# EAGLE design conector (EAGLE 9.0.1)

## Sheet 1 of 2: Board to Board Headers
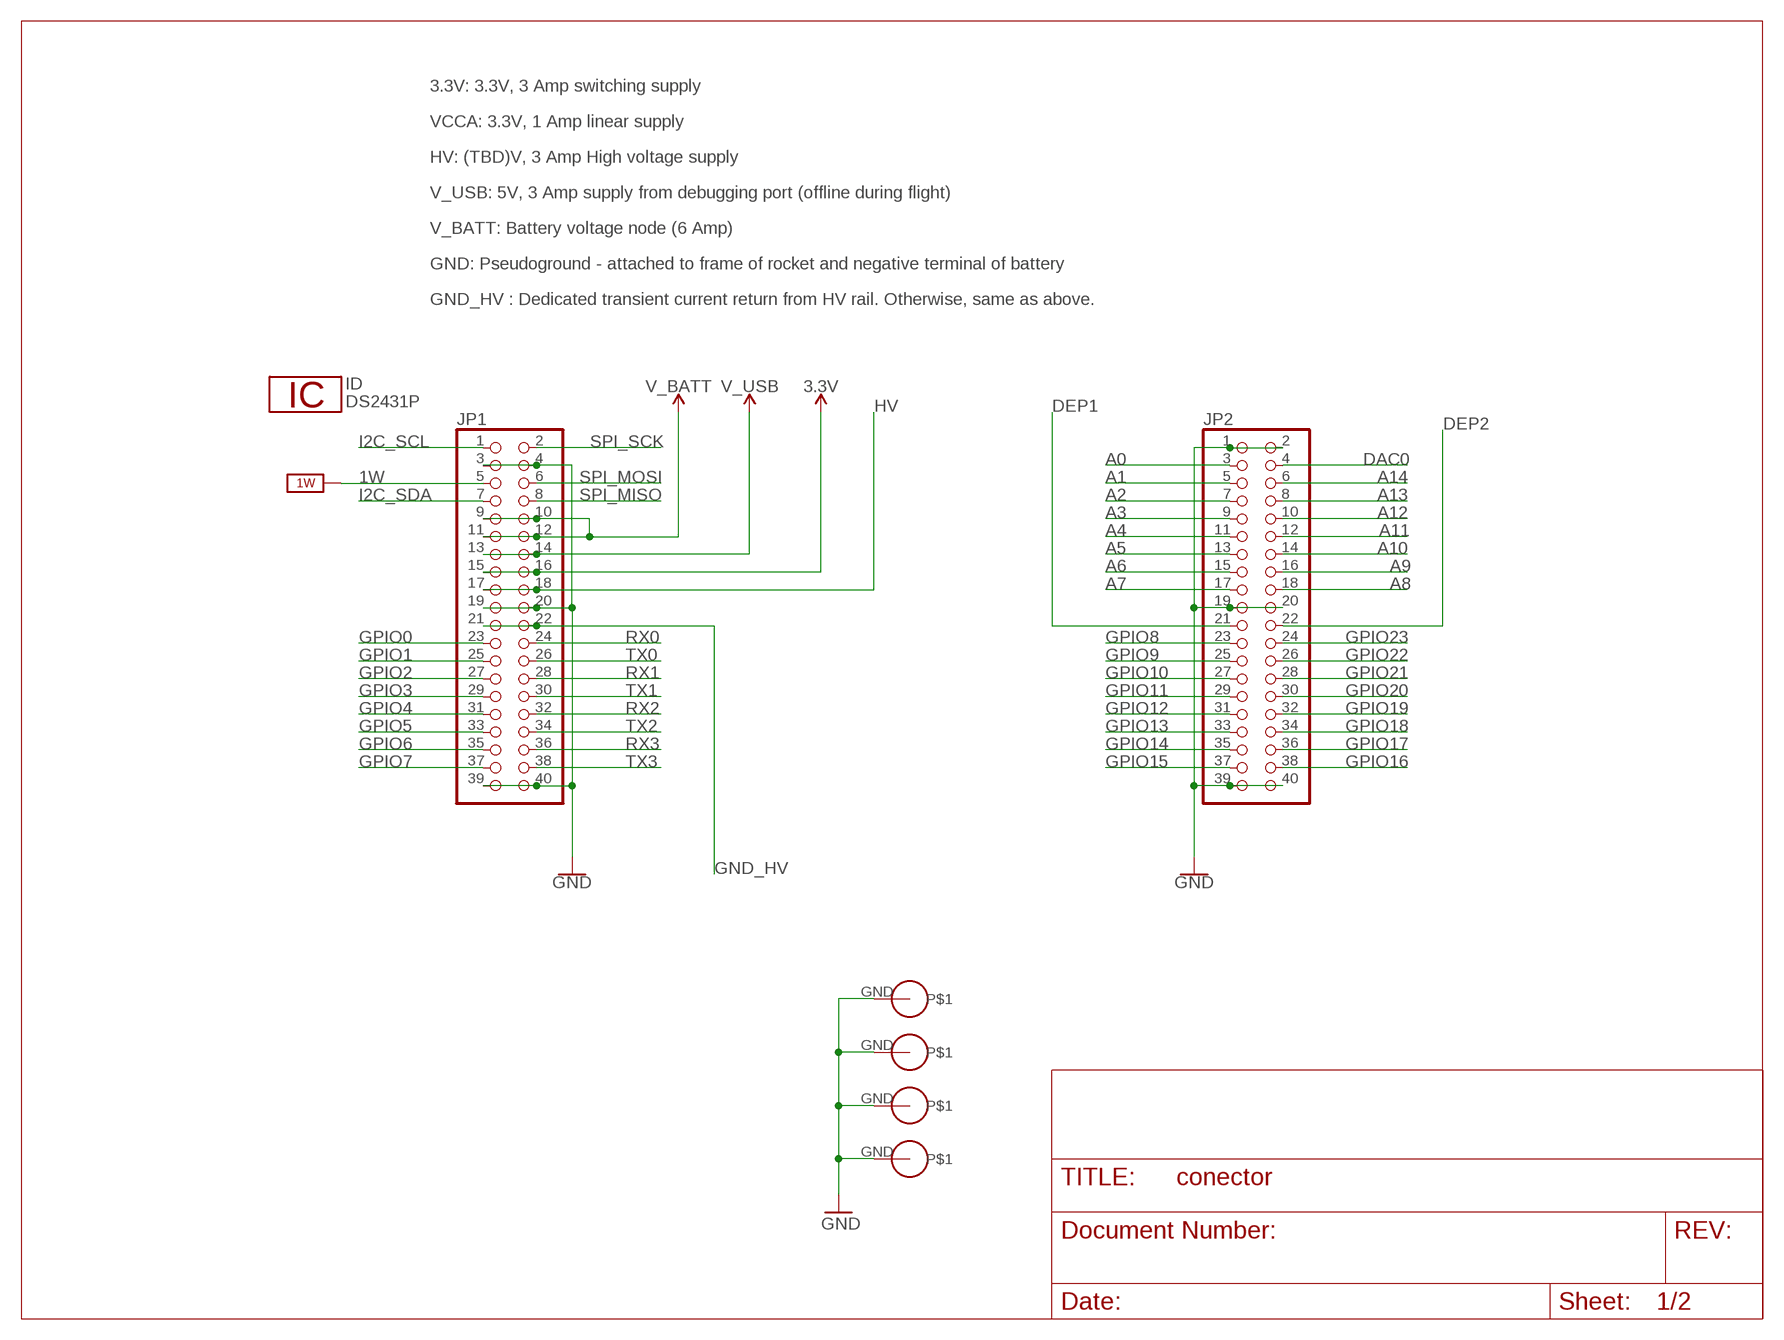
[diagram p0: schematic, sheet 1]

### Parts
ID  DS2431P  [TSOC6]
JP1  PINHD-2X20  [2X20]
JP2  PINHD-2X20  [2X20]
U$1  PS/104-MOUNTING-HOLE  [PC/104-MOUNTING-HOLE]
U$2  PS/104-MOUNTING-HOLE  [PC/104-MOUNTING-HOLE]
U$3  PS/104-MOUNTING-HOLE  [PC/104-MOUNTING-HOLE]
U$4  PS/104-MOUNTING-HOLE  [PC/104-MOUNTING-HOLE]

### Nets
1W: JP1.5 ; supply symbol labelled 1W_SUP
3.3V: JP1.15 JP1.16 ; also sheet 2
A0: JP2.3
A1: JP2.5
A2: JP2.7
A3: JP2.9
A4: JP2.11
A5: JP2.13
A6: JP2.15
A7: JP2.17
A8: JP2.18
A9: JP2.16
A10: JP2.14
A11: JP2.12
A12: JP2.10
A13: JP2.8
A14: JP2.6
DAC0: JP2.4
DEP1: JP2.21 ; also sheet 2
DEP2: JP2.22 ; also sheet 2
GND: JP1.3 JP1.4 JP1.19 JP1.20 JP1.39 JP1.40 JP2.1 JP2.2 JP2.19 JP2.20 JP2.39 JP2.40 U$1.GND U$2.GND U$3.GND U$4.GND ; also sheet 2
GND_HV: JP1.21 JP1.22 ; also sheet 2
GPIO0: JP1.23
GPIO8: JP2.23
GPIO9: JP2.25
GPIO10: JP2.27
GPIO11: JP2.29
GPIO12: JP2.31
GPIO13: JP2.33
GPIO14: JP2.35 ; also sheet 2
GPIO15: JP2.37 ; also sheet 2
GPIO16: JP2.38
GPIO17: JP2.36
GPIO18: JP2.34
GPIO19: JP2.32
GPIO20: JP2.30
GPIO21: JP2.28
GPIO22: JP2.26
GPIO23: JP2.24
HV: JP1.17 JP1.18
I2C_SCL: JP1.1
I2C_SDA: JP1.7
RX0: JP1.24
RX1: JP1.28
RX2: JP1.32
RX3: JP1.36
SPI_MISO: JP1.8
SPI_MOSI: JP1.6
SPI_SCK: JP1.2
TX0: JP1.26
TX1: JP1.30
TX2: JP1.34
TX3: JP1.38
V_BATT: JP1.9 JP1.10 JP1.11 JP1.12 ; also sheet 2
V_USB: JP1.13 JP1.14
Unconnected: JP1.25 JP1.27 JP1.29 JP1.31 JP1.33 JP1.35 JP1.37

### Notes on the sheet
- 3.3V: 3.3V, 3 Amp switching supply
- VCCA: 3.3V, 1 Amp linear supply
- HV: (TBD)V, 3 Amp High voltage supply
- V_USB: 5V, 3 Amp supply from debugging port (offline during flight)
- V_BATT: Battery voltage node (6 Amp)
- GND: Pseudoground - attached to frame of rocket and negative terminal of battery
- GND_HV : Dedicated transient current return from HV rail. Otherwise, same as above.

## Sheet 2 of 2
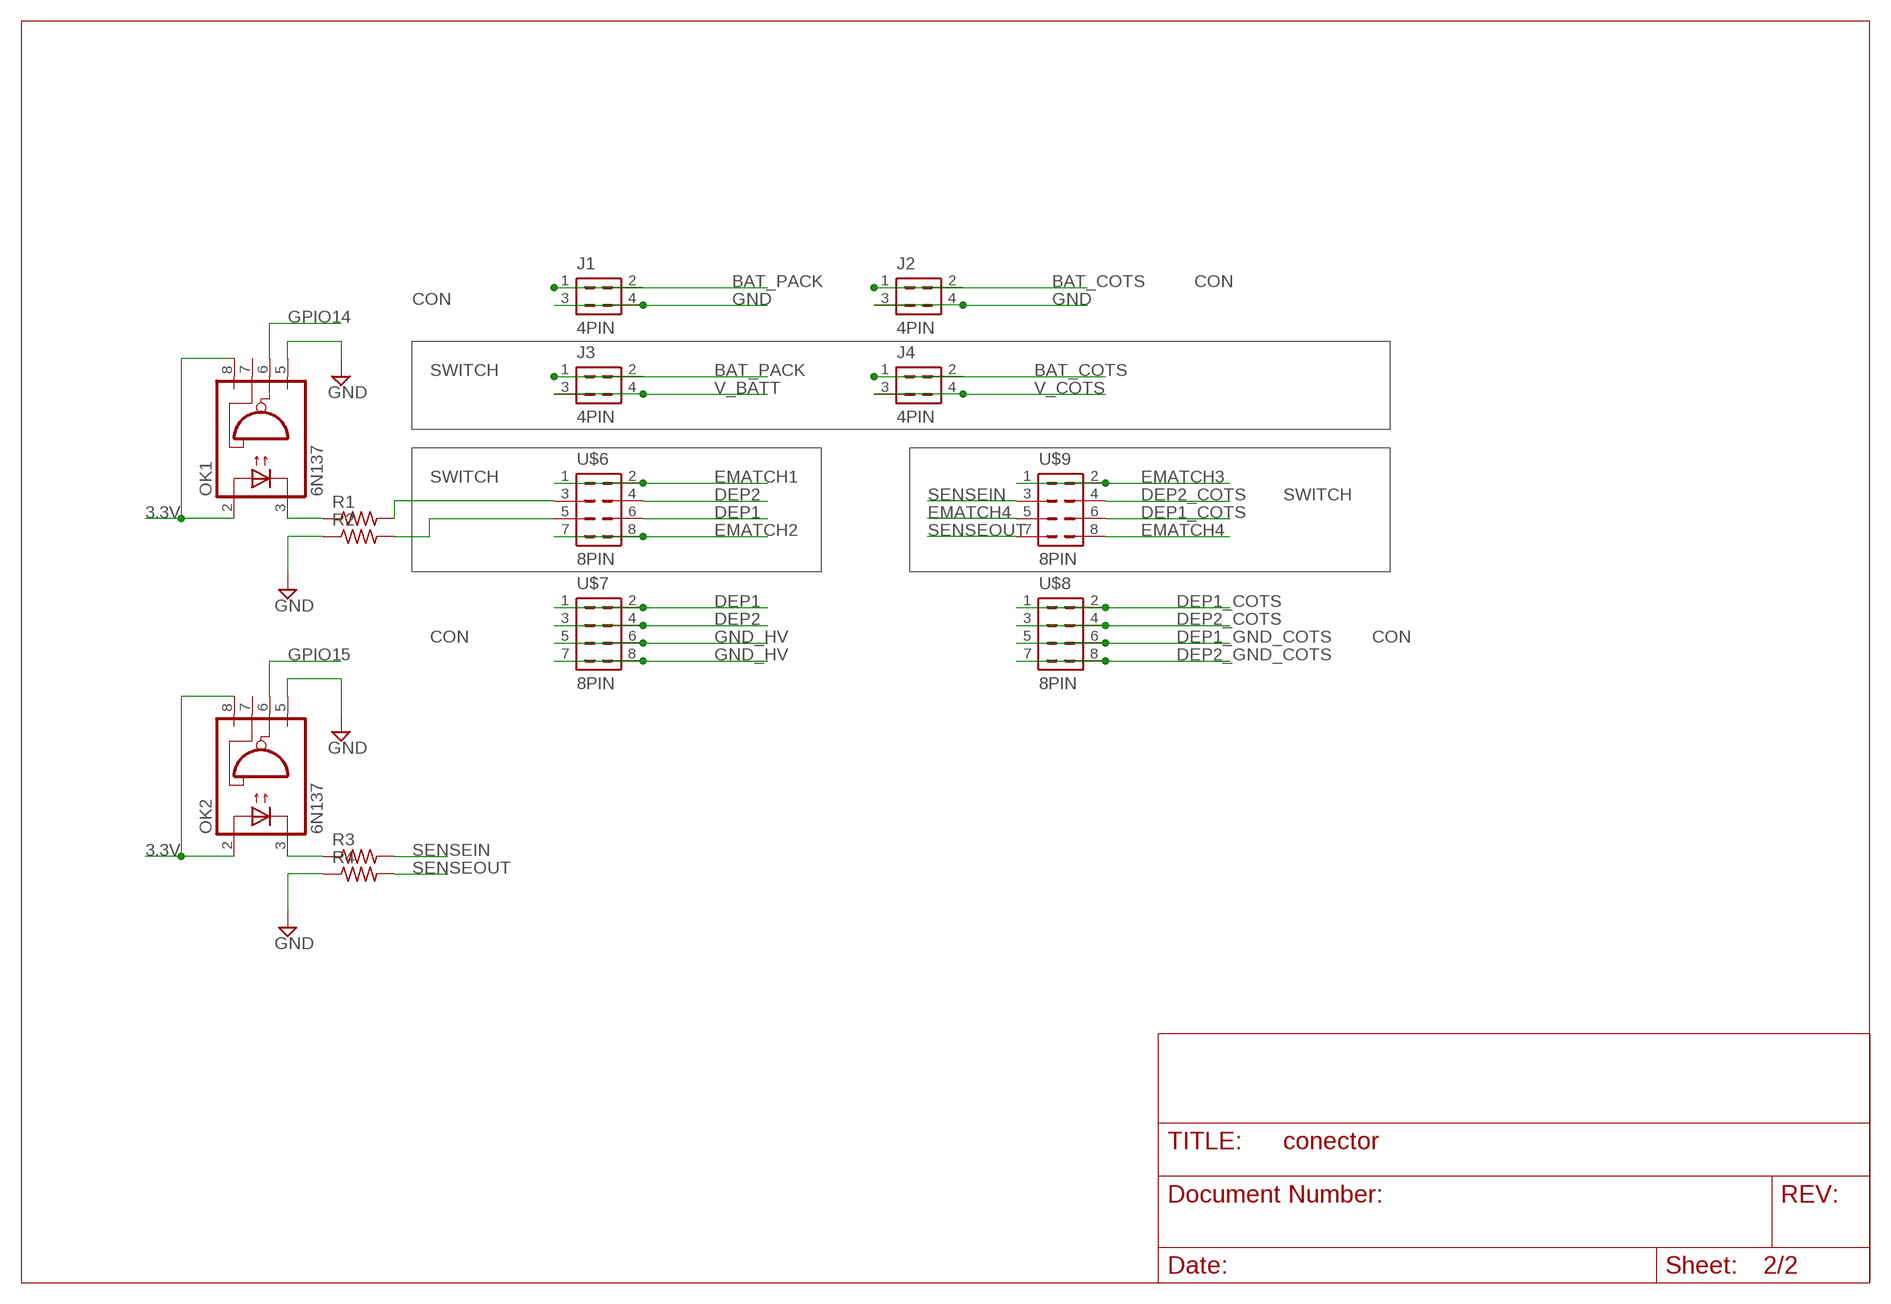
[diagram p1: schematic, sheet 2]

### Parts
J1  4PIN  [4PIN]
J2  4PIN  [4PIN]
J3  4PIN  [4PIN]
J4  4PIN  [4PIN]
OK1  6N137  [DIL08]
OK2  6N137  [DIL08]
R1  R-US_M1206  [M1206]
R2  R-US_M1206  [M1206]
R3  R-US_M1206  [M1206]
R4  R-US_M1206  [M1206]
U$6  8PIN  [8PIN]
U$7  8PIN  [8PIN]
U$8  8PIN  [8PIN]
U$9  8PIN  [8PIN]

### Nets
3.3V: OK1.2(A) OK1.8(VCC) OK2.2(A) OK2.8(VCC) ; also sheet 1
BAT_COTS: J2.1 J2.2 J4.1 J4.2
BAT_PACK: J1.1 J1.2 J3.1 J3.2
DEP1: U$6.6 U$7.1 U$7.2 ; also sheet 1
DEP1_COTS: U$8.1 U$8.2 U$9.6
DEP1_GND_COTS: U$8.5 U$8.6
DEP2: U$6.4 U$7.3 U$7.4 ; also sheet 1
DEP2_COTS: U$8.3 U$8.4 U$9.4
DEP2_GND_COTS: U$8.7 U$8.8
EMATCH1: U$6.1 U$6.2
EMATCH2: U$6.7 U$6.8
EMATCH3: U$9.1 U$9.2
EMATCH4: U$9.5 U$9.8
GND: J1.3 J1.4 J2.3 J2.4 OK1.5(GND) OK2.5(GND) R2.1 R4.1 ; also sheet 1
GND_HV: U$7.5 U$7.6 U$7.7 U$7.8 ; also sheet 1
GPIO14: OK1.6(VO) ; also sheet 1
GPIO15: OK2.6(VO) ; also sheet 1
N$1: OK1.3(C) R1.1
N$2: R1.2 U$6.3
N$3: R2.2 U$6.5
N$4: OK2.3(C) R3.1
SENSEIN: R3.2 U$9.3
SENSEOUT: R4.2 U$9.7
V_BATT: J3.3 J3.4 ; also sheet 1
V_COTS: J4.3 J4.4
Unconnected: OK1.7(VE) OK2.7(VE)

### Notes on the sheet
- CON
- CON
- SWITCH
- SWITCH
- SWITCH
- CON | CON

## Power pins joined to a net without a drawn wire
1W: ID.2(1W)
GND: ID.1(GND)

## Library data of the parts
ID = 1wire:DS2431: 1024-Bit EEPROM
J1-J4 = TOPCON:4PIN
JP1 JP2 = pinhead:PINHD-2X20: PIN HEADER
OK1 OK2 = optocoupler:6N137: MOTOROLA OPTO COUPLER; MPN: 6N137; OC_FARNELL: 1328376; OC_NEWARK: 52M1895
R1-R4 = rcl:R-US_: RESISTOR, American symbol; SPICEPREFIX: R
U$1-U$4 = CU inSpace 2019 Parts:PS/104-MOUNTING-HOLE: Mounting hole for PC/104 board.
U$6-U$9 = TOPCON:8PIN

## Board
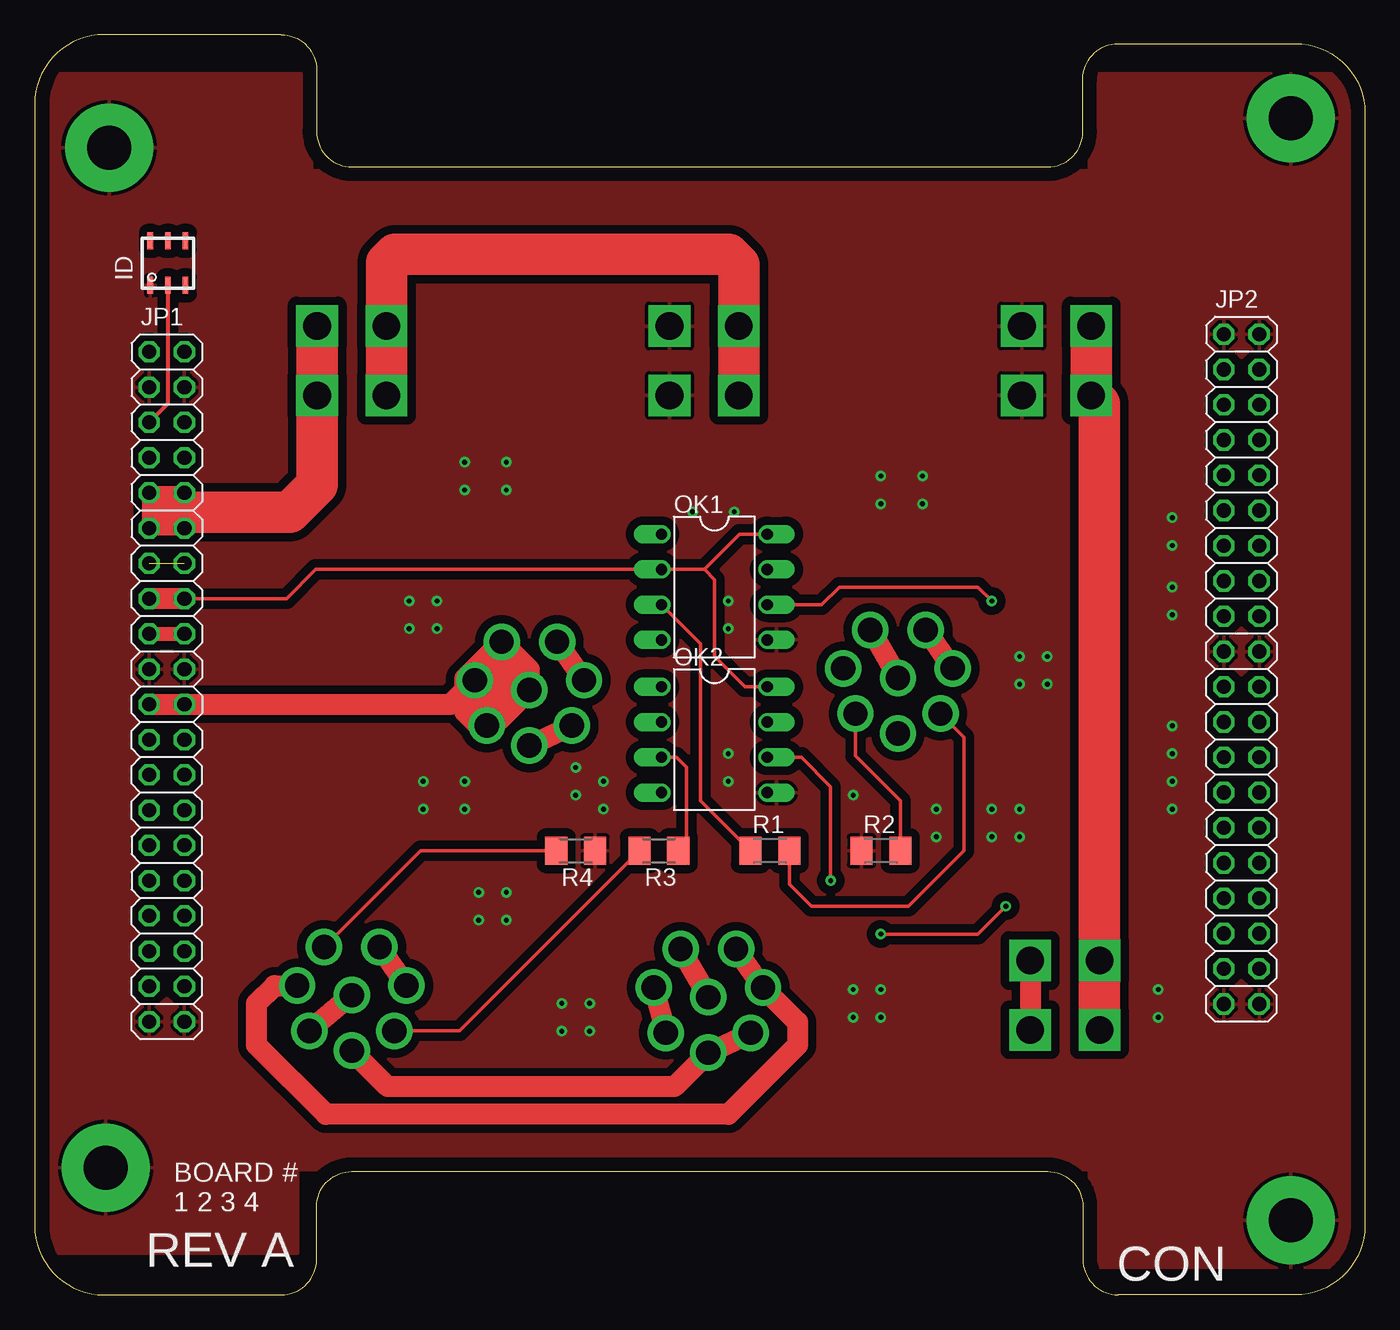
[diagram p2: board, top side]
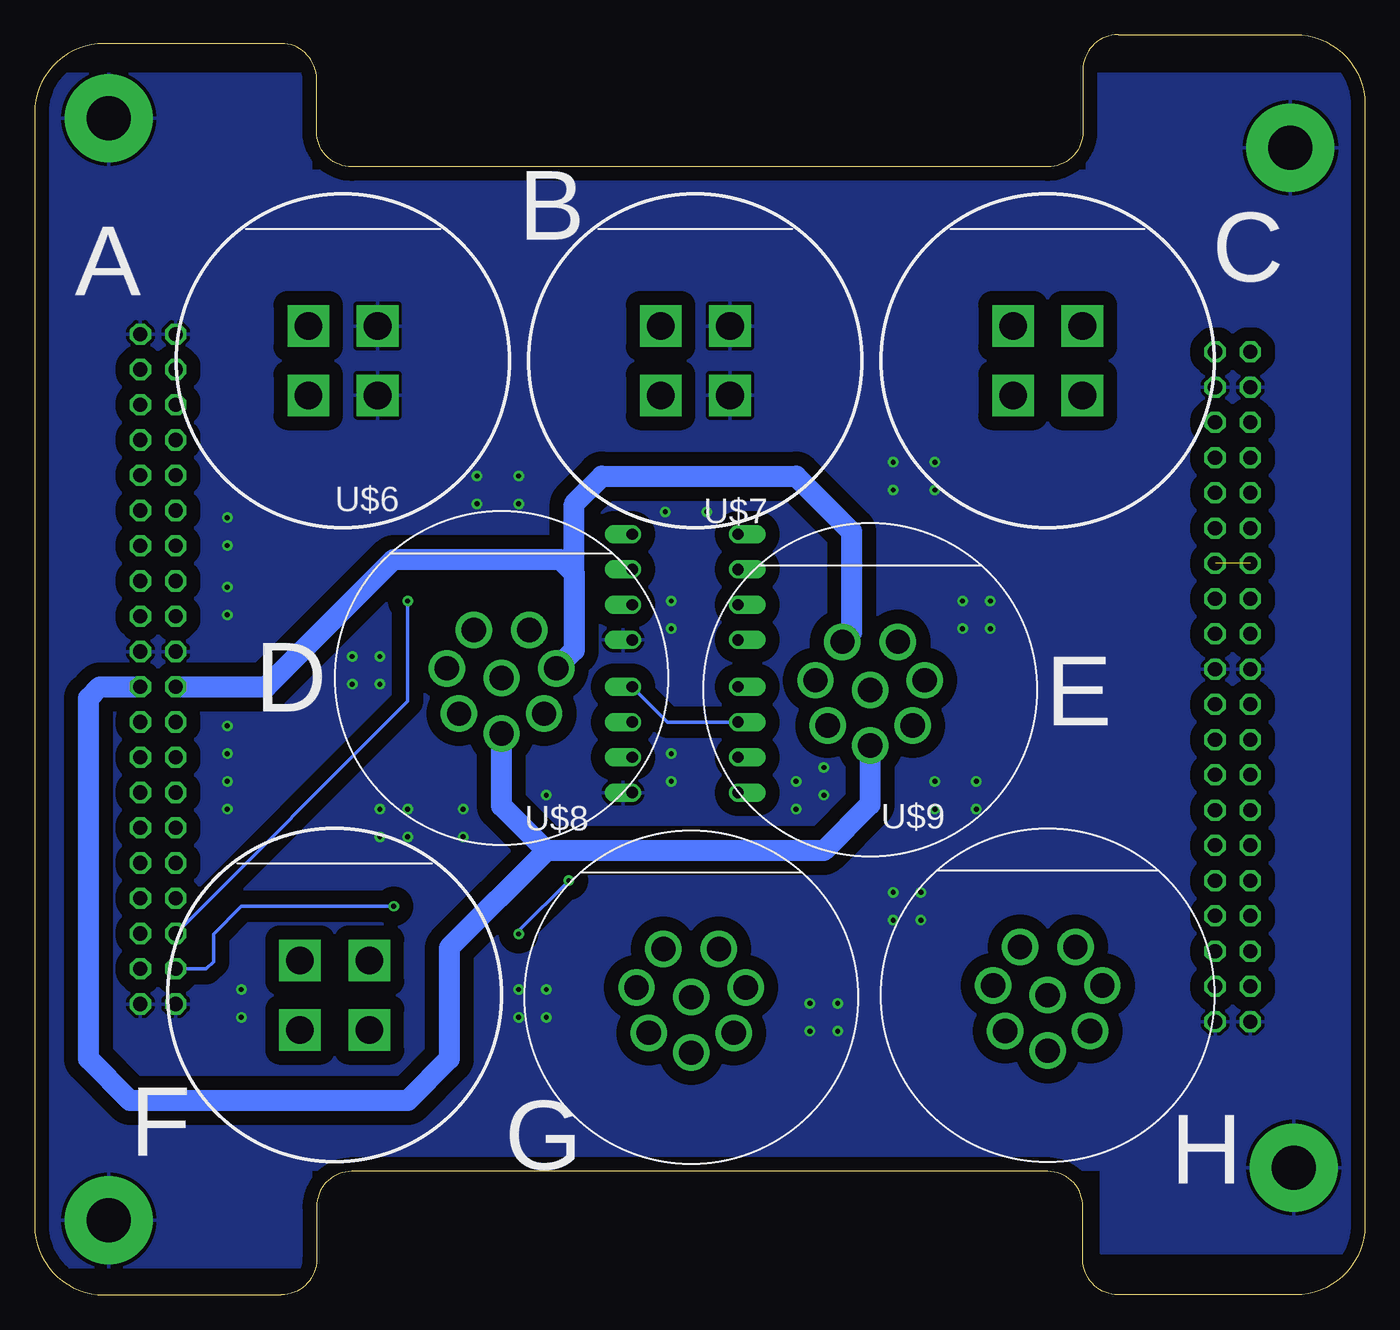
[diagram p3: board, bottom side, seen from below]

Size 95.89 x 90.81 mm. Coordinates in mm from the lower left corner, seen from the top.
Outline: 0,85.81 0,5 arc90 5,0 17.78,0 arc90 20.32,2.54 20.32,6.35 arc-90 22.86,8.89 73.03,8.89 arc-90 75.56,6.35 75.56,2.54 arc90 78.11,0 90.89,0 arc90 95.89,5 95.89,85.17 arc90 90.89,90.17 78.11,90.17 arc90 75.56,87.63 75.56,83.82 arc-90 73.03,81.28 22.86,81.28 arc-90 20.32,83.82 20.32,88.27 arc90 17.78,90.81 5,90.81 arc90 0,85.81
Copper layers (1*16): Top 0.035mm / dielectric 1.5mm / Bottom 0.035mm
Design rules "default": minimum track width 6mil, minimum drill 0.35mm, track to track 6mil, track to pad 6mil, pad to pad 6mil, via to via 6mil, smd to smd 6mil, copper to edge 40mil, drill to drill 6mil, minimum pad ring 10mil, minimum via ring 8mil, stop-mask expansion 4mil, vias tented up to drill 0mil, thermal gap 10mil

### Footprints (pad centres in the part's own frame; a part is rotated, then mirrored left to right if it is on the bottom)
TSOC6 = smd 0.406 x 1.219: 1 -1.27,-1.6; 2 0,-1.6; 3 1.27,-1.6; 4 1.27,1.6; 5 0,1.6; 6 -1.27,1.6
4PIN = drill 2 square: 1 -2.5,2.5; 2 -2.5,-2.5; 3 2.5,-2.5; 4 2.5,2.5
2X20 = drill 1.016 octagon: 1 -24.13,-1.27; 2 -24.13,1.27; 3 -21.59,-1.27; 4 -21.59,1.27; 5 -19.05,-1.27; 6 -19.05,1.27; 7 -16.51,-1.27; 8 -16.51,1.27; 9 -13.97,-1.27; 10 -13.97,1.27; 11 -11.43,-1.27; 12 -11.43,1.27; 13 -8.89,-1.27; 14 -8.89,1.27; 15 -6.35,-1.27; 16 -6.35,1.27; 17 -3.81,-1.27; 18 -3.81,1.27; 19 -1.27,-1.27; 20 -1.27,1.27; 21 1.27,-1.27; 22 1.27,1.27; 23 3.81,-1.27; 24 3.81,1.27; 25 6.35,-1.27; 26 6.35,1.27; 27 8.89,-1.27; 28 8.89,1.27; 29 11.43,-1.27; 30 11.43,1.27; 31 13.97,-1.27; 32 13.97,1.27; 33 16.51,-1.27; 34 16.51,1.27; 35 19.05,-1.27; 36 19.05,1.27; 37 21.59,-1.27; 38 21.59,1.27; 39 24.13,-1.27; 40 24.13,1.27
DIL08 = drill 0.813 offset: 1 -3.81,-3.81; 2 -1.27,-3.81; 3 1.27,-3.81; 4 3.81,-3.81; 5 3.81,3.81; 6 1.27,3.81; 7 -1.27,3.81; 8 -3.81,3.81
M1206 = smd 1.6 x 2: 1 -1.4,0; 2 1.4,0
PC/104-MOUNTING-HOLE = drill 3.175 pad 6.35: GND 0,0
8PIN = drill 1.75: 1 -2,3.464; 2 -3.939,0.695; 3 -3.064,-2.571; 4 0,-4; 5 3.064,-2.571; 6 3.939,0.695; 7 2,3.464; 8 0,0

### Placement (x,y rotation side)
ID  9.6,74.35 0 top
J1  48.26,67.31 0 bottom
J2  73.66,67.31 0 bottom
J3  22.86,67.31 0 bottom
J4  74.26,21.59 0 bottom
JP1  9.53,43.81 270 top
JP2  87,45.09 270 top
OK1  49,51 270 top
OK2  49,40 270 top
R1  53,32 0 top
R2  61,32 0 top
R3  45,32 180 top
R4  39,32 180 top
U$1  5.36,82.65 0 top
U$2  90.55,84.79 0 top
U$3  5.13,9.17 0 top
U$4  90.55,5.36 0 top
U$6  62.23,44.45 0 bottom
U$7  35.66,43.59 0 bottom
U$8  48.56,21.45 0 bottom
U$9  22.86,21.59 0 bottom

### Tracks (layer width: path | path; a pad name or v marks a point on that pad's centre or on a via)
1W
  Top 0.305: ID.2 9.6,64.21 JP1.5
3.3V
  Top 0.254: OK1.8 50.81,54.81 48.27,52.27 | 48.27,52.27 OK1.2 20.27,52.27 18.16,50.16 JP1.16 | 48.27,52.27 49,51.54 49,46 51.19,43.81 OK2.8
  Top 1.016: JP1.16 10.79,50.13
  Top 1.5: JP1.16 JP1.15
  Bottom 0.254: OK2.8 50.27,41.27 OK2.2
BAT_COTS
  Top 3: J4.2 J4.1 76.76,64.21 J2.2 J2.1
BAT_PACK
  Top 3: J1.2 J1.1 50.76,74.24 50,75 26,75 25.36,74.36 J3.1 J3.2
DEP1
  Top 1.5: U$7.1 U$7.2
  Bottom 1.5: JP2.21 79.19,43.81 70,53 58,53 57,52 | U$6.6 57,46.44 57,52 | 57,52 57,57 55,59 41,59 37,55 37,47.71 U$7.1
DEP1_COTS
  Top 1.5: U$9.6 17.29,22.29 16,21 16,18 21,13 50,13 55,18 55,19.64 U$8.2 U$8.1
DEP1_GND_COTS
  Top 1.5: U$8.6 U$8.5
DEP2
  Top 1.5: U$7.4 U$7.3
  Bottom 1.5: U$7.4 35.66,35.34 39,32 59,32 | U$6.4 62.23,35.23 59,32 | 59,32 66,25 66,17 69,14 89,14 92,17 92,43 91.19,43.81 JP2.22
DEP2_COTS
  Top 1.5: U$9.4 25.45,15 46.11,15 U$8.4 U$8.3
DEP2_GND_COTS
  Top 1.5: U$8.7 U$8.8
EMATCH1
  Top 1.5: U$6.1 U$6.2
EMATCH2
  Top 1.5: U$6.7 U$6.8
EMATCH3
  Top 1.5: U$9.2 U$9.1
EMATCH4
  Top 1.5: U$9.8 U$9.5
GND  (via drill 0.35)
  other vias: 81,22 81,20 71,35 71,33 69,35 69,33 73,46 73,44 71,46 71,44 82,37 82,35 82,41 82,39 82,51 82,49 82,56 82,54 61,22 61,20 59,22 59,20 40,21 40,19 38,21 38,19 32,29 32,27 34,29 34,27 41,37 41,35 39,38 39,36 31,37 31,35 28,37 28,35 29,50 29,48 27,50 27,48 34,60 34,58 31,60 31,58 61,59 61,57 64,59 64,57 65,35 65,33 50,39 50,37 50,50 50,48 50.43,56.42 47.43,56.42 59,36
  pour Top (isolate 0.61): 1,11 1,3 19,3 19,9 76,9 76,2 96,2 96,87 96,88 76,88 76,81 20,81 20,88 1,88
  pour Bottom (isolate 1.016): 1,88 1,3 19,3 19,9 76,9 76,2 96,2 96,88 76,88 76,81 20,81 20,88
GND_HV
  Top 1.5: JP1.21 JP1.22 29.98,42.55 U$7.6 | U$7.6 31.72,41.89 U$7.5 | U$7.5 33.09,41.02 U$7.8 | U$7.8 35.66,45.05 U$7.7 | U$7.7 31.72,45.12 U$7.6 | U$7.6 32.41,43.59 U$7.8 | U$7.7 31,44.39 31,42 31.98,41.02 U$7.5 | U$7.5 32.6,44.6 33,45 34,45 35,44 34,43 33,43 32.6,42.6 U$7.5
GPIO14  (via drill 0.35)
  Top 0.254: v69,50 68,51 58,51 56.73,49.73 OK1.6
  Bottom 0.254: JP2.35 69,42.76 v69,50
GPIO15  (via drill 0.35)
  Top 0.254: OK2.6 55.27,38.73 57.38,36.62 v57.38,29.84 | v61,26 68,26 v70,28
  Bottom 0.254: v57.38,29.84 61,26.22 v61,26 | v70,28 81,28 83,26 83,24 83.5,23.5 JP2.37
HV
  Top 1.016: JP1.17 JP1.18
N$1
  Top 0.254: R1.1 48,35.6 48,46.92 OK1.3
N$2
  Top 0.254: R1.2 54.4,29.6 56,28 63,28 67,32 67,40.17 U$6.3
N$3
  Top 0.254: U$6.5 59.17,38.83 62.4,35.6 R2.2
N$4
  Top 0.254: R3.1 47,32.6 47,38 46.27,38.73 OK2.3
SENSEIN
  Top 0.254: U$9.3 30.62,19.02 R3.2
SENSEOUT
  Top 0.254: R4.2 27.81,32 U$9.7
V_BATT
  Top 1.016: 9,55.24 JP1.11 JP1.9 | 9,55.24 10,55.24 | 10,55.24 JP1.12 JP1.10 10,57.78 | JP1.9 10,57.78 | JP1.9 9,57.78 9,55.24 | 10,55.24 10,56.39 10,57.78
  Top 3: J3.4 J3.3 20.36,58.36 18.39,56.39 10,56.39
V_COTS
  Top 1.5: J4.4 J4.3
V_USB  (1 unrouted)

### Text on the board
tPlace: BOARD # / 1 2 3 4 | REV A | CON
bPlace: B | C | A | D | E | F | G | H

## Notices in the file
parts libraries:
SparkFun-PowerSymbols: Licensing: Creative Commons ShareAlike 4.0 International - https://creativecommons.org/licenses/by-sa/4.0
